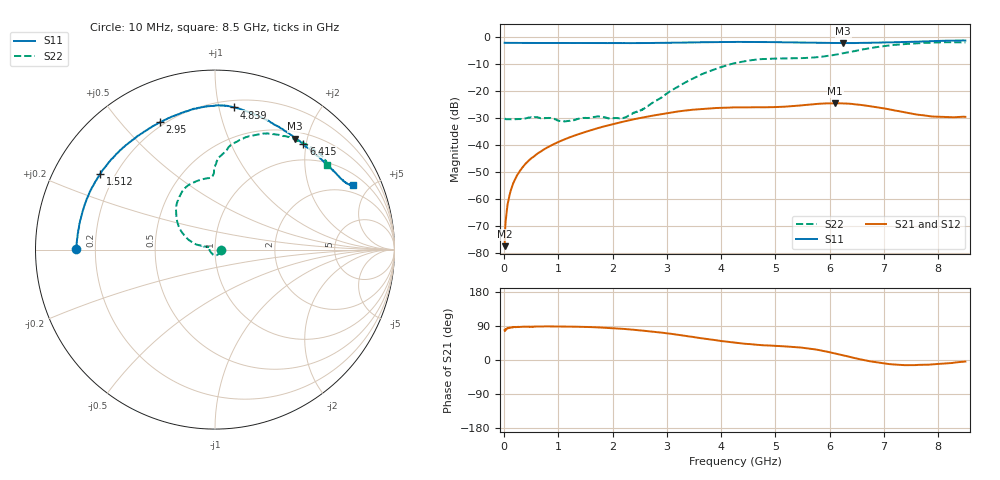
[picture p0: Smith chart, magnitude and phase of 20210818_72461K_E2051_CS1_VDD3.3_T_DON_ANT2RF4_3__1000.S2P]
!Agilent Technologies,E5071C,MY46417908,A.11.23
!Date: Wed Aug 18 14:32:49 2021
!Data & Calibration Information:
!Freq	S11:SOLT2(ON)	S21:SOLT2(ON)	S12:SOLT2(ON)	S22:SOLT2(ON)
!PortZ  Port1:50+j0  Port2:50+j0
!Above PortZ is port z conversion or system Z0 setting when saving the data.
!When reading, reference impedance value at option line is always used.
# Hz S dB R 50
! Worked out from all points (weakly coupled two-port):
!   1601 points, 10 MHz to 8.5 GHz, reference 50 ohm
!   highest |S21| = -24.59 dB at 6.102 GHz (marker M1); lowest = -77.5 dB at 10 MHz (marker M2)
!   lowest |S11| = -2.3 dB at 6.25 GHz (marker M3), VSWR 7.44, Z = 30.4 + j89.9 ohm
!   |S11| at or under -10 dB: nowhere
!   |S22| runs from -31.4 to -2.0 dB; largest |S21 - S12| = 0.00026
!   S11 on the Smith chart (normalised r, x): 10 MHz: 0.13, +0.00; 1.512 GHz: 0.14, +0.29; 2.95 GHz: 0.18, +0.64; 4.839 GHz: 0.25, +1.11; 6.415 GHz: 0.68, +1.95; 8.5 GHz: 1.51, +3.95
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1e7  -2.21 179.7  -77.52 79.0  -76.59 82.8  -30.22 -2.2
6.30625e7  -2.25 178.5  -62.25 84.3  -62.39 83.4  -30.53 -6.9
1.108188e8  -2.25 177.4  -57.80 84.7  -57.95 85.4  -30.51 -11.4
2.063312e8  -2.27 175.2  -52.57 86.9  -52.52 87.0  -30.47 -22.6
3.28375e8  -2.28 172.5  -48.67 87.7  -48.62 87.9  -30.43 -39.4
7.581812e8  -2.30 162.8  -41.42 88.8  -41.43 88.8  -30.09 -92.9
1.097781e9  -2.30 155.5  -38.12 88.5  -38.13 88.4  -31.31 -136.9
1.426769e9  -2.31 148.5  -35.69 87.4  -35.70 87.4  -30.14 -177.1
1.511669e9  -2.31 146.6  -35.16 87.3  -35.16 87.2  -30.09 176.4
2.206788e9  -2.33 131.2  -31.38 82.0  -31.38 81.9  -30.01 155.4
2.843538e9  -2.26 115.8  -28.84 73.2  -28.84 73.0  -23.18 164.4
2.949662e9  -2.24 113.4  -28.46 71.3  -28.45 71.4  -21.74 163.7
3.634169e9  -2.04 99.5  -26.74 57.4  -26.73 57.5  -13.95 153.3
4.255e9  -1.91 89.9  -26.14 45.7  -26.15 45.8  -9.76 131.5
4.838688e9  -1.95 82.3  -26.10 38.4  -26.10 38.4  -8.16 110.2
5.671769e9  -2.20 67.7  -25.04 29.3  -25.04 29.5  -7.70 91.8
6.101575e9  -2.29 57.8  -24.59 17.2  -24.62 17.2  -6.64 90.0
6.25015e9  -2.35 54.1  -24.70 12.3  -24.71 12.3  -6.09 88.6
6.414644e9  -2.30 50.0  -24.87 6.6  -24.89 6.6  -5.48 85.6
7.088538e9  -2.06 35.5  -26.84 -10.6  -26.88 -10.8  -3.24 68.8
8.017131e9  -1.52 25.5  -29.60 -10.4  -29.60 -10.4  -2.08 44.0
8.5e9  -1.40 25.1  -29.65 -4.0  -29.69 -4.4  -2.13 37.2
